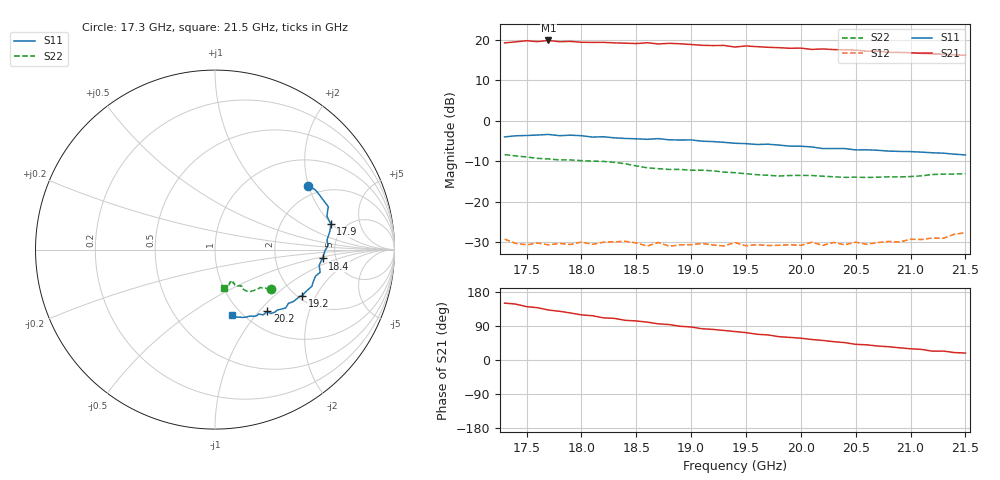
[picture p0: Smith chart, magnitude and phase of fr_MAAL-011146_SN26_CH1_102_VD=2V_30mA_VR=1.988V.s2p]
!Typical measured data - probed
!Date: Friday, August 19, 2022 11:56:10
!Correction: S11(Full 2 Port(1,2))
!S21(Full 2 Port(1,2))
!S12(Full 2 Port(1,2))
!S22(Full 2 Port(1,2))
!S2P File: Measurements: S11, S21, S12, S22:
# Hz S  dB  R 50
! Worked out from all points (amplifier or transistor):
!   43 points, 17.3 GHz to 21.5 GHz, reference 50 ohm
!   highest |S21| = 19.8 dB at 17.7 GHz (marker M1)
!   |S21| within 3 dB of that: start of sweep to 20.97 GHz
!   unconditionally stable (mu >= 1): start of sweep to end of sweep
!   at 18 GHz: K = 1.09, MAG = 22.8 dB, |S12| = -30.0 dB
!   at 19.4 GHz: K = 1.54, MAG = 19.8 dB, |S12| = -30.1 dB
!   at 21.5 GHz: K = 1.70, MAG = 17.0 dB, |S12| = -27.7 dB
!   S11 on the Smith chart (normalised r, x): 17.3 GHz: 1.69, +1.99; 17.9 GHz: 3.86, +1.95; 18.4 GHz: 3.92, -0.61; 19.2 GHz: 2.12, -1.56; 20.2 GHz: 1.29, -1.11; 21.5 GHz: 0.90, -0.76
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1.73e10  -4.03 34.4  19.19 150.1  -29.28 -46.0  -8.40 -35.5
1.74e10  -3.75 31.0  19.44 147.6  -30.32 -48.3  -8.72 -36.7
1.75e10  -3.68 29.1  19.72 140.8  -30.67 -42.4  -8.99 -37.2
1.76e10  -3.57 24.6  19.50 138.1  -30.23 -47.4  -9.33 -38.7
1.77e10  -3.42 20.8  19.79 131.9  -30.67 -43.3  -9.46 -39.3
1.79e10  -3.60 12.4  19.56 124.1  -30.60 -45.0  -9.72 -41.8
1.8e10  -3.73 9.5  19.35 119.0  -29.99 -44.8  -9.89 -42.9
1.83e10  -4.26 -0.6  19.19 109.9  -29.93 -48.2  -10.30 -49.9
1.84e10  -4.42 -4.7  19.12 104.7  -29.81 -43.9  -10.66 -52.4
1.86e10  -4.63 -8.6  19.23 100.0  -30.98 -48.0  -11.66 -54.8
1.87e10  -4.45 -12.2  18.92 95.4  -30.10 -47.5  -11.87 -53.7
1.88e10  -4.75 -14.8  19.09 93.5  -31.01 -48.3  -12.07 -54.2
1.92e10  -5.19 -27.7  18.53 80.7  -30.71 -50.3  -12.41 -57.6
1.94e10  -5.60 -33.2  18.16 75.0  -30.12 -52.9  -12.87 -60.7
1.95e10  -5.69 -34.3  18.43 72.3  -30.91 -51.3  -13.12 -60.3
1.98e10  -6.04 -41.5  18.01 61.5  -30.79 -49.3  -13.69 -60.9
2.01e10  -6.51 -49.0  17.58 54.1  -30.04 -52.2  -13.56 -62.9
2.02e10  -6.91 -49.6  17.70 51.6  -30.81 -52.1  -13.73 -63.7
2.05e10  -7.24 -55.6  17.41 41.3  -30.03 -52.3  -13.96 -64.3
2.08e10  -7.53 -61.8  16.84 35.0  -29.85 -52.6  -13.88 -65.6
2.12e10  -7.95 -70.1  16.45 23.3  -29.00 -53.8  -13.32 -68.8
2.15e10  -8.48 -75.6  16.17 18.3  -27.69 -57.1  -13.15 -77.4
